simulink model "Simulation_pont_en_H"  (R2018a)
settings: Solver=FixedStepAuto  StartTime=0.0  StopTime=0.1  MaxStep=Ts  RelTol=1e-3
PreLoadFcn:
  | Ts=1/60/3240;
InitFcn:
  | Ts=1/60/3240;
libraries: powerlib x8

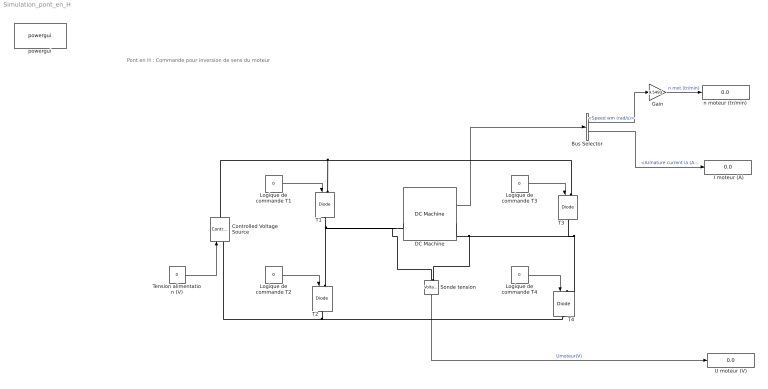
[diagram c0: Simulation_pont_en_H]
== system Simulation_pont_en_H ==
  note: Pont en H : Commande pour inversion de sens du moteur
  " I moteur (A)" : Display
  Bus Selector : BusSelector  OutputSignals=Speed wm (rad/s),Armature current ia (A)
  Controlled Voltage Source : powerlib/Electrical Sources/Controlled Voltage Source  Initialize=on  Source_Type=DC  Amplitude=0  Phase=0  Frequency=0  Measurements=None
  DC Machine : powerlib/Machines/DC Machine  PresetModel=No  MechanicalLoad=Torque TL  FieldType=Permanent magnet  ShowDetailedParameters=on  MeasurementBus=off  RLa="[ 0.6  0.0012]"  RLf="[ 240  120]"  Laf=1.8  MachineConstant=Back-emf constant (V/rpm)  Ke=6.31579E-4  Kt=1.8  J=1e-8  Bm=0  Tf=0.00045  w0=1  Ifinit=1  TsPowergui=0  TsBlock=-1
  Gain : Gain  Gain=9.5493
  Logique de commande T{1..4} (4 alike) : Constant  Value=0
  Sonde tension : powerlib/Measurements/Voltage Measurement  Tag=PoWeRsYsTeMmEaSuReMeNt  PhasorSimulation=off  OutputType=Magnitude  PSBequivalent=0
  T{1..4} (4 alike) : powerlib/Power Electronics/IGBT//Diode  Ron=1e-3  Rs=1e5  Cs=inf  Measurements=off
  Tension alimentation (V) : Constant  Value=0
  U moteur (V) : Display
  n moteur (tr/min) : Display
  powergui : powerlib/powergui  SimulationMode=Discrete  SampleTime=Ts  frequency=60  Iterations=50  frequencyindice=0  Pbase=100e6  ErrMax=1e-4  UnitsV=kV  UnitsW=MW  buscounter=0  FunctionMessages=off  echomessages=off  EnableUseOfTLC=off  CurrentSourceSwitches=off  DisableSnubberDevices=off  DisableRonSwitches=off  DisableVfSwitches=off  DisplayEquations=off  SolverType=Tustin/Backward Euler (TBE)  Interpol=off  ExternalGateDelay=off  methode=off  Ts=100  x0status=blocks  SPID=off  SwTol=0  HookPort=off  RestoreLinks=warning  ResistiveCurrentMeasurement=off  Frange=[0:2:500]  Ylog=off  Xlog=on  ShowGrid=off  save=off  variable=ZData  structure=sps1phPWM1_str  ZoomFFT=on  StartTime=0.1-2/60  cycles=2  DisplayStyle=1  fundamental=60  FreqAxis=off  MaxFrequency=5000  frequencyindicesteady=1  RmsSteady=1  display=off
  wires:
  Sonde tension/1 -> U moteur (V)/1  "Umoteur(V)"
  Tension alimentation (V)/1 -> Controlled Voltage Source/1
  Logique de commande T1/1 -> T1/1
  Logique de commande T4/1 -> T4/1
  Logique de commande T3/1 -> T3/1
  Logique de commande T2/1 -> T2/1
  DC Machine/1 -> Bus Selector/1
  Bus Selector/1 -> Gain/1  "<Speed wm (rad/s)>"
  Bus Selector/2 -> " I moteur (A)"/1  "<Armature current ia (A)>"
  Gain/1 -> n moteur (tr/min)/1  "n mot (tr/min)"
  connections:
  T2/RConn1 -- T4/RConn1 -- Controlled Voltage Source/LConn1
  T3/LConn1 -- T1/LConn1 -- Controlled Voltage Source/RConn1
  T1/RConn1 -- Sonde tension/LConn1 -- DC Machine/LConn1 -- T2/LConn1
  Sonde tension/LConn2 -- DC Machine/RConn1 -- T3/RConn1 -- T4/LConn1
